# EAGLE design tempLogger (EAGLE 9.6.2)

## Sheet 1 of 4: ESP32 Connections
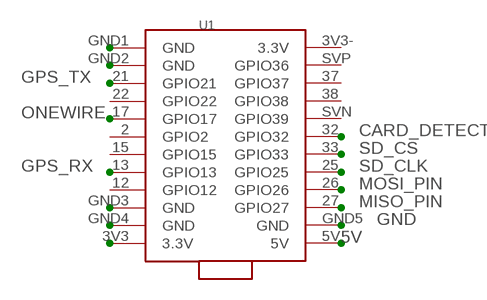
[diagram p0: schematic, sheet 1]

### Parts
U1  ESP32-TTGO  [ESP32-TTGO-TDISPLAY]

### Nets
3V3: U1.3V3(3.3V)
5V: U1.5V ; also sheet 2,3,4
CARD_DETECT: U1.32(GPIO32) ; also sheet 3
GND: U1.GND1(GND) U1.GND2(GND) U1.GND3(GND) U1.GND4(GND) U1.GND5(GND) ; also sheet 2,3,4
GPS_RX: U1.13(GPIO13) ; also sheet 4
GPS_TX: U1.21(GPIO21) ; also sheet 4
MISO_PIN: U1.27(GPIO27) ; also sheet 3
MOSI_PIN: U1.26(GPIO26) ; also sheet 3
ONEWIRE: U1.17(GPIO17) ; also sheet 2
SD_CLK: U1.25(GPIO25) ; also sheet 3
SD_CS: U1.33(GPIO33) ; also sheet 3
Unconnected: U1.2(GPIO2) U1.3V3-(3.3V) U1.12(GPIO12) U1.15(GPIO15) U1.22(GPIO22) U1.37(GPIO37) U1.38(GPIO38) U1.SVN(GPIO39) U1.SVP(GPIO36)

## Sheet 2 of 4: ONEWIRE Bus Connections
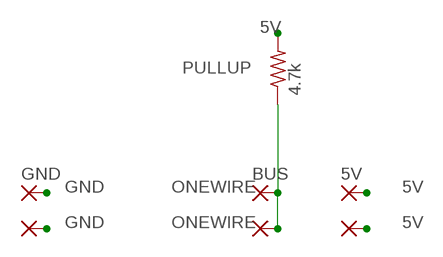
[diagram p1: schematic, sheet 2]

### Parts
5V  SMD5  [SMD2,54-5,08]
BUS  SMD5  [SMD2,54-5,08]
GND  SMD5  [SMD2,54-5,08]
GND$1  SMD5  [SMD2,54-5,08]
PAD5  SMD5  [SMD2,54-5,08]
PAD6  SMD5  [SMD2,54-5,08]
PULLUP  4.7k  R-US_0204/7  [0204/7]

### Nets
5V: 5V.1(P) PAD6.1(P) PULLUP.2 ; also sheet 1,3,4
GND: GND$1.1(P) GND.1(P) ; also sheet 1,3,4
ONEWIRE: BUS.1(P) PAD5.1(P) PULLUP.1 ; also sheet 1

## Sheet 3 of 4: Micro SD Reader Connections
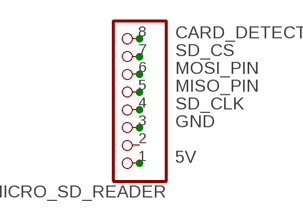
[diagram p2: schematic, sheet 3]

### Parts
MICRO_SD_READER  PINHD-1X8  [1X08]

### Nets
5V: MICRO_SD_READER.1 ; also sheet 1,2,4
CARD_DETECT: MICRO_SD_READER.8 ; also sheet 1
GND: MICRO_SD_READER.3 ; also sheet 1,2,4
MISO_PIN: MICRO_SD_READER.5 ; also sheet 1
MOSI_PIN: MICRO_SD_READER.6 ; also sheet 1
SD_CLK: MICRO_SD_READER.4 ; also sheet 1
SD_CS: MICRO_SD_READER.7 ; also sheet 1
Unconnected: MICRO_SD_READER.2

## Sheet 4 of 4: GPS Module Connections
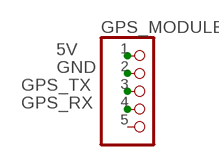
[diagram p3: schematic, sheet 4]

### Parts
GPS_MODULE  PINHD-1X5  [1X05]

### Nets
5V: GPS_MODULE.1 ; also sheet 1,2,3
GND: GPS_MODULE.2 ; also sheet 1,2,3
GPS_RX: GPS_MODULE.4 ; also sheet 1
GPS_TX: GPS_MODULE.3 ; also sheet 1
Unconnected: GPS_MODULE.5

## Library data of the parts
5V BUS GND GND$1 PAD5 PAD6 = wirepad:SMD5: SMD PAD
GPS_MODULE = pinhead:PINHD-1X5: PIN HEADER
MICRO_SD_READER = pinhead:PINHD-1X8: PIN HEADER
PULLUP = adafruit:R-US_: RESISTOR, American symbol
U1 = EPS32_TTGO_TDISPLAY:ESP32-TTGO: ESP32-TTGO-T Display ESP32 Breakout board with an inbuild OLED display

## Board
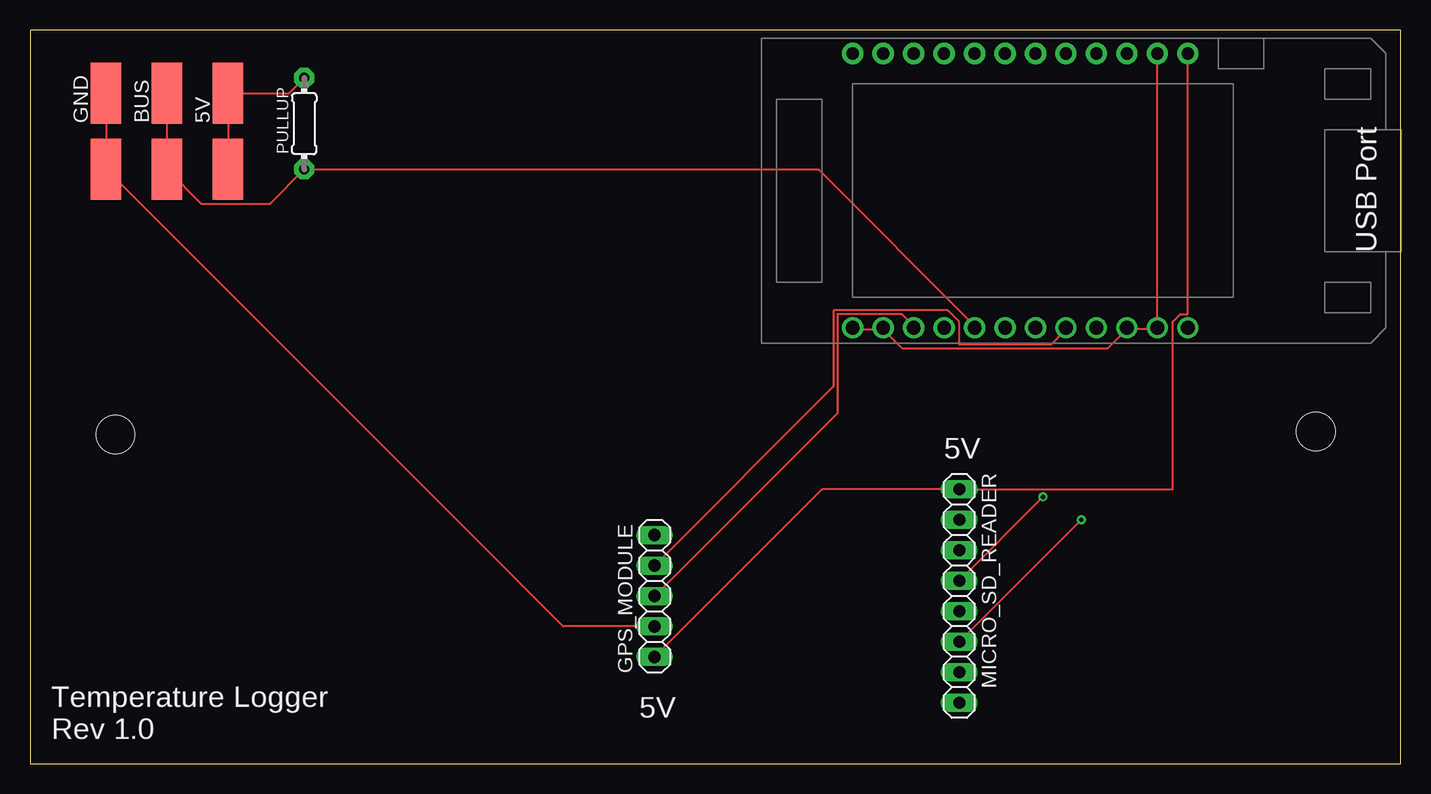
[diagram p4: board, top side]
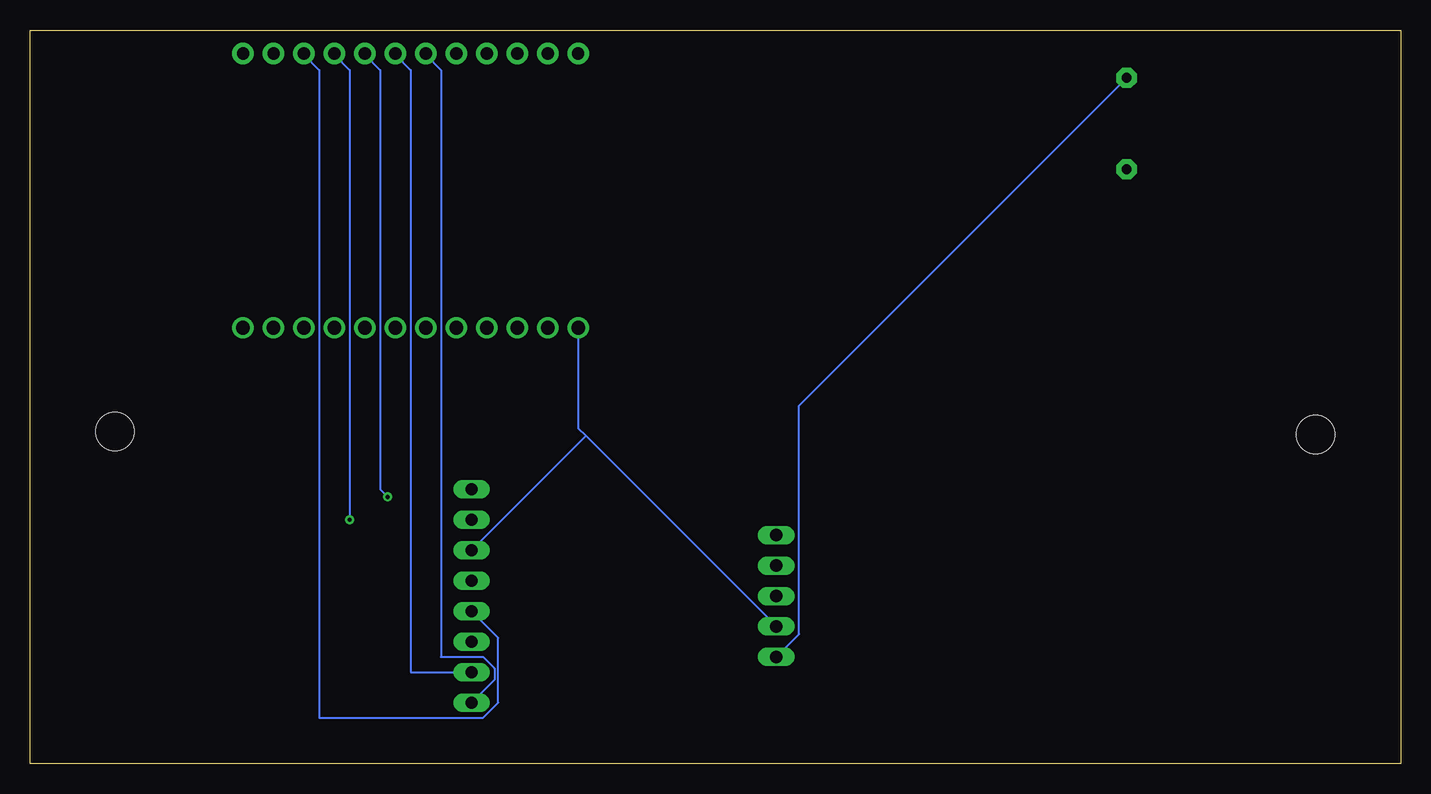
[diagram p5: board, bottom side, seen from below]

Size 114.28 x 61.14 mm. Coordinates in mm from the lower left corner, seen from the top.
Outline: 0,0 114.28,0 114.28,61.14 0,61.14 0,0
Copper layers (1*16): Top 0.035mm / dielectric 1.5mm / Bottom 0.035mm
Design rules "default": minimum track width 6mil, minimum drill 0.35mm, track to track 6mil, track to pad 6mil, pad to pad 6mil, via to via 6mil, smd to smd 6mil, copper to edge 40mil, drill to drill 6mil, minimum pad ring 10mil, minimum via ring 8mil, stop-mask expansion 4mil, vias tented up to drill 0mil, thermal gap 10mil
Holes 3.2 mm at 7.11,27.43 107.19,27.69

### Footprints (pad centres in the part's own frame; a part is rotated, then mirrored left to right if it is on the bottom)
SMD2,54-5,08 = smd 2.54 x 5.08: 1 0,0
1X05 = drill 1.016 long: 1 -5.08,0; 2 -2.54,0; 3 0,0; 4 2.54,0; 5 5.08,0
1X08 = drill 1.016 long: 1 -8.89,0; 2 -6.35,0; 3 -3.81,0; 4 -1.27,0; 5 1.27,0; 6 3.81,0; 7 6.35,0; 8 8.89,0
0204/7 = drill 0.813 pad 1.676 octagon: 1 -3.81,0; 2 3.81,0
ESP32-TTGO-TDISPLAY = drill 1.143 pad 1.778: 2 0,15.24; 3V3 0,0; 12 0,7.62; 13 0,10.16; 15 0,12.7; 17 0,17.78; 21 0,22.86; 22 0,20.32; GND1 0,27.94; GND2 0,25.4; GND3 0,5.08; GND4 0,2.54 | drill 1.016 pad 1.778: 3V3- 22.86,27.94; 5V 22.86,0; 25 22.86,10.16; 26 22.86,7.62; 27 22.86,5.08; 32 22.86,15.24; 33 22.86,12.7; 37 22.86,22.86; 38 22.86,20.32; GND5 22.86,2.54; SVN 22.86,17.78; SVP 22.86,25.4

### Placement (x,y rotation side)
5V  16.51,55.88 0 top
BUS  11.43,55.88 0 top
GND  6.35,55.88 0 top
GND$1  6.35,49.53 0 top
GPS_MODULE  52.07,13.97 90 top
MICRO_SD_READER  77.47,13.97 270 top
PAD5  11.43,49.53 0 top
PAD6  16.51,49.53 0 top
PULLUP  22.86,53.34 90 top
U1  96.52,36.32 90 top

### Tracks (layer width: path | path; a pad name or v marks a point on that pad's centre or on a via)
5V
  Top 0.152: PULLUP.2 21.59,55.88 5V.1 PAD6.1 | GPS_MODULE.1 66.04,22.86 MICRO_SD_READER.1 95.25,22.86 95.25,36.83 95.89,37.46 96.52,37.46 U1.5V
  Bottom 0.152: PULLUP.2 50.16,29.85 50.16,10.8 GPS_MODULE.1
CARD_DETECT
  Bottom 0.152: MICRO_SD_READER.8 75.56,6.98 75.56,7.94 76.52,8.89 80.01,8.89 80.01,57.79 81.28,59.05 U1.32
GND
  Top 0.152: 91.44,36.2 93.98,36.2 U1.GND4 U1.GND5 | GND.1 GND$1.1 44.45,11.43 GPS_MODULE.2 | 71.12,36.2 68.58,36.2 U1.GND1 | 91.44,36.2 89.85,34.61 72.71,34.61 71.12,36.2 | 91.44,36.2 U1.GND3 | 71.12,36.2 U1.GND2
  Bottom 0.152: 67.94,27.3 68.58,27.94 U1.GND1 | 67.94,27.3 GPS_MODULE.2 | 67.94,27.3 MICRO_SD_READER.3
GPS_RX
  Top 0.152: GPS_MODULE.4 66.99,31.43 66.99,37.78 76.52,37.78 77.47,36.83 77.47,34.93 85.09,34.93 86.36,36.2 U1.13
GPS_TX
  Top 0.152: GPS_MODULE.3 67.31,29.21 67.31,37.46 72.71,37.46 73.66,36.51 U1.21
MISO_PIN
  Bottom 0.152: MICRO_SD_READER.5 75.25,10.48 75.25,5.08 76.52,3.81 90.17,3.81 90.17,57.79 91.44,59.05 U1.27
MOSI_PIN  (via drill 0.35)
  Top 0.152: v87.63,20.32 MICRO_SD_READER.6
  Bottom 0.152: v87.63,20.32 87.63,57.79 88.9,59.05 U1.26
ONEWIRE
  Top 0.152: U1.17 78.74,36.51 65.72,49.53 PULLUP.1 20,46.67 14.29,46.67 PAD5.1 BUS.1
SD_CLK  (via drill 0.35)
  Top 0.152: v84.46,22.23 MICRO_SD_READER.4
  Bottom 0.152: v84.46,22.23 85.09,22.86 85.09,57.79 86.36,59.05 U1.25
SD_CS
  Bottom 0.152: MICRO_SD_READER.7 82.55,7.62 82.55,57.79 83.82,59.05 U1.33

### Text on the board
tPlace: USB Port | 5V | 5V | Temperature Logger / Rev 1.0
